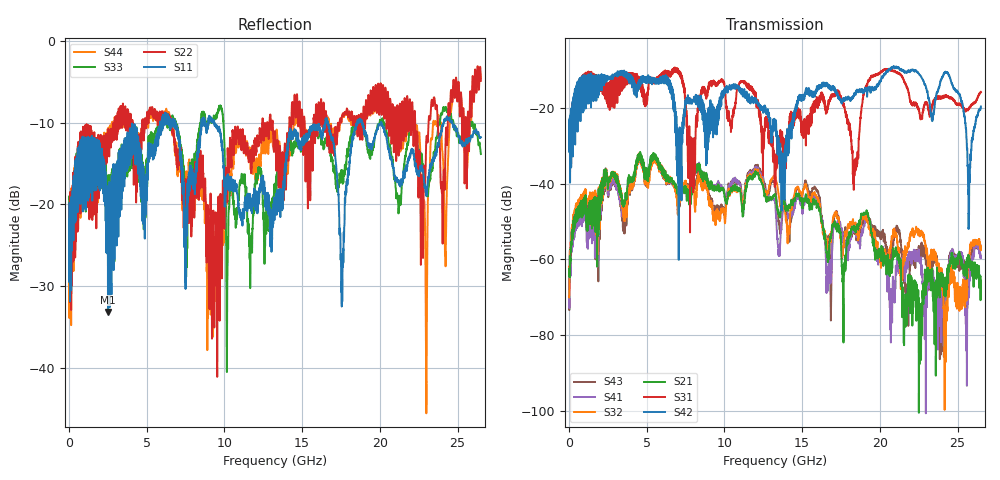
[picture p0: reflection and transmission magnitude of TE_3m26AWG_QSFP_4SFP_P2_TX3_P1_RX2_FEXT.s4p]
!Agilent Technologies,N5222A,MY51421691,A.10.00.00
!Agilent N5222A: A.10.00.00
!Date: Friday, January 30, 2015 12:36:44
!Correction: S11(Full 4 Port(1,2,3,4))
!S12(Full 4 Port(1,2,3,4))
!S13(Full 4 Port(1,2,3,4))
!S14(Full 4 Port(1,2,3,4))
!S21(Full 4 Port(1,2,3,4))
!S22(Full 4 Port(1,2,3,4))
!S23(Full 4 Port(1,2,3,4))
!S24(Full 4 Port(1,2,3,4))
!S31(Full 4 Port(1,2,3,4))
!S32(Full 4 Port(1,2,3,4))
!S33(Full 4 Port(1,2,3,4))
!S34(Full 4 Port(1,2,3,4))
!S41(Full 4 Port(1,2,3,4))
!S42(Full 4 Port(1,2,3,4))
!S43(Full 4 Port(1,2,3,4))
!S44(Full 4 Port(1,2,3,4))
!S4P File: Measurements: <S11,S12,S13,S14>,
!<S21,S22,S23,S24>,
!<S31,S32,S33,S34>,
!<S41,S42,S43,S44>:
# Hz S  dB  R 50.0
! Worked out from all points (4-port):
!   2650 points, 10 MHz to 26.5 GHz, reference 50 ohm
!   strongest paths, dB at 10 MHz, 6.63 GHz, 13.26 GHz, 19.88 GHz, 26.5 GHz:
!     S42: -24.7, -16.1, -25.2, -13.9, -19.6
!     S31: -24.9, -10.4, -34.1, -10.8, -15.7
!     S21: -62.5, -39.2, -42.8, -58.5, -65.7
!     S32: -70.1, -39.7, -38.0, -59.5, -56.6
!     S41: -66.0, -39.5, -44.7, -59.9, -59.3
!     S43: -65.9, -39.8, -40.4, -53.9, -56.8
!   lowest |S11| = -33.2 dB at 2.51 GHz (marker M1), VSWR 1.04, Z = 51 - j1.95 ohm
!   |S11| at or under -10 dB: start of sweep to 5.869 GHz; 9.355 GHz to 16.5 GHz (7.142 GHz wide, 55.3 % of centre); 20.09 GHz to 24.1 GHz (4.004 GHz wide, 18.1 % of centre)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
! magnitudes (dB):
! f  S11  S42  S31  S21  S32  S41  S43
! 10 MHz  -19.9  -24.7  -24.9  -62.5  -70.1  -66.0  -65.9
! 2.51 GHz  -33.2  -12.3  -19.7  -40.7  -40.7  -42.0  -41.8
! 13.77 GHz  -17.8  -33.6  -31.7  -45.2  -45.5  -45.8  -46.3
! 15.33 GHz  -12.2  -16.2  -23.4  -45.1  -41.7  -44.8  -40.6
! 22.94 GHz  -18.1  -14.0  -18.7  -69.4  -56.6  -73.3  -58.7
! 25.74 GHz  -12.0  -48.3  -20.1  -61.8  -60.0  -69.1  -62.3
! 26.5 GHz  -11.8  -19.6  -15.7  -65.7  -56.6  -59.3  -56.8
